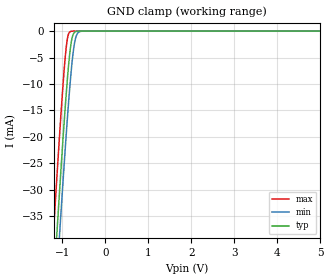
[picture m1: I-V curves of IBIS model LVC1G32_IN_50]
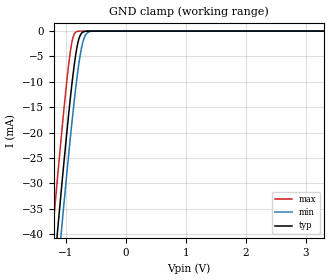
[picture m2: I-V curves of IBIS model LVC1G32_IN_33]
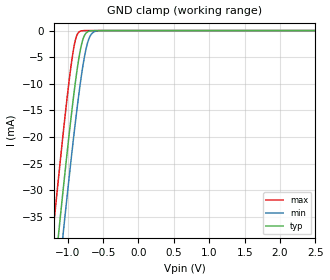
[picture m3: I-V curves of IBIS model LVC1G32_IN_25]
| TEXAS INSTRUMENTS INCORPORATED
| Standard Linear and Logic Group
| IBIS Model of SN74LVC1G32
| SINGLE 2-INPUT POSITIVE-OR GATE
| This file contains package information for the following:
|  SON 6-pin (DSF) package as [Component] LVC1G32_DSF
|  SOT 5-pin (DBV) package as [Component] LVC1G32_DBV
|  SOT 5-pin (DCK) package as [Component] LVC1G32_DCK
|  USON 6-pin (DRY) package as [Component] LVC1G32_DRY
|  NanoStar WCSP 5-pin (YEA) package as [Component] LVC1G32_YEA
|  NanoFree WCSP 5-pin (YZA) package as [Component] LVC1G32_YZA
|  NanoStar WCSP 5-pin (YEP) package as [Component] LVC1G32_YEP
|  NanoFree WCSP 5-pin (YZP) package as [Component] LVC1G32_YZP
| This device can be powered at the following Vccs:
|  5.0 volt Vcc
|  3.3 volt Vcc
|  2.5 volt Vcc
|  1.8 volt Vcc
| This file provides unique models under the [Model Selector] for each Vcc.
| For operation at a specific Vcc, select the appropriate model after each
| [Model Selector] keyword.
[IBIS Ver]   3.2
[Comment char]  |_char
[File Name]   sn74lvc1g32.ibs
[File Rev]   1.4 | d_die
[Date]   03/06/2014
[Source]
| Texas Instruments Incorporated.
| Analog-eLab Design Center, HPA
| 12500 TI Blvd
| Dallas, TX -75243
[Notes]   Revision History:
| The following is an IBIS list for the SN74LVC1G07.
| Please contact sllibis@ti.com with questions and
| comments concerning SLL IBIS models.
| - FILE REV HISTORY
| - 1.4 DSF package added 03/06/2014.
| - Rev 1.3. Added package component LVC1G32_DRY
| - 1.2 YEA, YEP, YZA, and YZP packages added on 05/18/04
| - As there is no power clamp diode in the Input Model,
|   we removed the Pwr Clamp table data from those Models.
| - Due to the fact that the Device is 5-V Input/Output
|   tolarent, the Model has some Non-Monotonic Warnings.
[Disclaimer]
| This model is designed as an aid for customers of Texas Instruments
| TI and its licensors and suppliers make no warranties, either expressed
| or implied, with respect to this  model, including the warranties of
| merchantability or fitness for a particular purpose.
| The model is provided solely on an "as is" basis. The entire risk as to
| its quality and performance is with the customer.
[Copyright]
(C) Copyright 2014 Texas Instruments Incorporated.All rights reserved.
| Component LVC1G32_DSF 6-pin SON
[Component]   LVC1G32_DSF
[Manufacturer]   Texas Instruments, Inc.
[Package]
|   typ   min   max
R_pkg   0.04185   0.03442   0.04904
L_pkg   0.42366nH   0.34696nH   0.51073nH
C_pkg   0.11042pF   0.10608pF   0.11529pF
[Pin]   signal_name   model_name   R_pin   L_pin   C_pin
1   A   LVC1G32_IN   0.04209   0.41329nH   0.10991pF
2   B   LVC1G32_IN   0.03442   0.34696nH   0.10608pF
3   GND   GND   0.04429   0.45885nH   0.11207pF
4   Y   LVC1G32_OUT   0.04904   0.51073nH   0.11529pF
5   nc   nc   0.00037   0.03788nH   0.07652pF
6   VCC   POWER   0.04377   0.44894nH   0.11182pF
| Component LVC1G32_DBV 5-pin SOT
[Component]   LVC1G32_DBV
[Manufacturer]   Texas Instruments, Inc.
[Package]
|   typ   min   max
R_pkg   2.500e-02   2.100e-02   2.900e-02
L_pkg   1.529e-09   1.312e-09   1.906e-09
C_pkg   1.560e-13   1.100e-13   2.400e-13
[Pin]   signal_name   model_name   R_pin   L_pin   C_pin
1   A   LVC1G32_IN   2.100e-02   1.511e-09   1.440e-13
2   B   LVC1G32_IN   2.300e-02   1.312e-09   1.380e-13
3   GND   GND   2.900e-02   1.906e-09   2.400e-13
4   Y   LVC1G32_OUT   2.600e-02   1.541e-09   1.500e-13
5   VCC   POWER   2.500e-02   1.374e-09   1.100e-13
| Component LVC1G32_DCK 5-pin SOT
[Component]   LVC1G32_DCK
[Manufacturer]   Texas Instruments, Inc.
[Package]
|   typ   min   max
R_pkg   2.000e-02   1.700e-02   2.500e-02
L_pkg   9.980e-10   8.810e-10   1.069e-09
C_pkg   1.460e-13   1.180e-13   2.050e-13
[Pin]   signal_name   model_name   R_pin   L_pin   C_pin
1   A   LVC1G32_IN   1.900e-02   1.069e-09   1.620e-13
2   B   LVC1G32_IN   1.800e-02   8.810e-10   1.210e-13
3   GND   GND   1.700e-02   1.031e-09   2.050e-13
4   Y   LVC1G32_OUT   2.000e-02   9.600e-10   1.240e-13
5   VCC   POWER   2.500e-02   1.049e-09   1.180e-13
| Component LVC1G32_YEA 5-pin NanoStar WCSP
[Component]   LVC1G32_YEA
[Manufacturer]   Texas Instruments, Inc.
[Package]
|   typ   min   max
R_pkg   0.001   0.001   0.001
L_pkg   0.021nH   0.021nH   0.021nH
C_pkg   0.046pF   0.045pF   0.047pF
[Pin]   signal_name   model_name   R_pin   L_pin   C_pin
1   A   LVC1G32_IN   0.001   0.021nH   0.046pF
2   B   LVC1G32_IN   0.001   0.021nH   0.047pF
3   GND   GND   0.001   0.021nH   0.046pF
4   Y   LVC1G32_OUT   0.001   0.021nH   0.045pF
5   VCC   POWER   0.001   0.021nH   0.045pF
| Component LVC1G32_YZA 5-pin NanoFree WCSP
[Component]   LVC1G32_YZA
[Manufacturer]   Texas Instruments, Inc.
[Package]
|   typ   min   max
R_pkg   0.001   0.001   0.001
L_pkg   0.021nH   0.021nH   0.021nH
C_pkg   0.046pF   0.045pF   0.047pF
[Pin]   signal_name   model_name   R_pin   L_pin   C_pin
1   A   LVC1G32_IN   0.001   0.021nH   0.046pF
2   B   LVC1G32_IN   0.001   0.021nH   0.047pF
3   GND   GND   0.001   0.021nH   0.046pF
4   Y   LVC1G32_OUT   0.001   0.021nH   0.045pF
5   VCC   POWER   0.001   0.021nH   0.045pF
| Component LVC1G32_YEP 5-pin NanoStar WCSP
[Component]   LVC1G32_YEP
[Manufacturer]   Texas Instruments, Inc.
[Package]
|   typ   min   max
R_pkg   0.001   0.001   0.001
L_pkg   0.021nH   0.021nH   0.021nH
C_pkg   0.046pF   0.045pF   0.047pF
[Pin]   signal_name   model_name   R_pin   L_pin   C_pin
1   A   LVC1G32_IN   0.001   0.021nH   0.046pF
2   B   LVC1G32_IN   0.001   0.021nH   0.047pF
3   GND   GND   0.001   0.021nH   0.046pF
4   Y   LVC1G32_OUT   0.001   0.021nH   0.045pF
5   VCC   POWER   0.001   0.021nH   0.045pF
| Component LVC1G32_YZP 5-pin NanoFree WCSP
[Component]   LVC1G32_YZP
[Manufacturer]   Texas Instruments, Inc.
[Package]
|   typ   min   max
R_pkg   0.001   0.001   0.001
L_pkg   0.021nH   0.021nH   0.021nH
C_pkg   0.046pF   0.045pF   0.047pF
[Pin]   signal_name   model_name   R_pin   L_pin   C_pin
1   A   LVC1G32_IN   0.001   0.021nH   0.046pF
2   B   LVC1G32_IN   0.001   0.021nH   0.047pF
3   GND   GND   0.001   0.021nH   0.046pF
4   Y   LVC1G32_OUT   0.001   0.021nH   0.045pF
5   VCC   POWER   0.001   0.021nH   0.045pF
| Component LVC1G32_DRY 6-pin USON
[Component]   LVC1G32_DRY
[Manufacturer]   Texas Instruments, Inc.
[Package]
|   typ   min   max
R_pkg   0.04988   0.00103   0.05683
L_pkg   0.40631n   0.01445n   0.47858n
C_pkg   0.10742p   0.07652p   0.11194p
[Pin]   signal_name   model_name   R_pin   L_pin   C_pin
1   A   LVC1G32_IN   0.05683   0.47858n   0.11194p
2   A   LVC1G32_IN   0.04686   0.38124n   0.10769p
3   GND   GND   0.05415   0.45213n   0.10986p
4   Y   LVC1G32_OUT   0.05132   0.42056n   0.10715p
5   NC   NC   0.00103   0.01445n   0.07652p
6   VCC   POWER   0.04843   0.39205n   0.10505p
| Model LVC1G32_IN
[Model Selector]   LVC1G32_IN
LVC1G32_IN_50   5.0 volt Vcc
LVC1G32_IN_33   3.3 volt Vcc
LVC1G32_IN_25   2.5 volt Vcc
LVC1G32_IN_18   1.8 volt Vcc
| Model LVC1G32_OUT
[Model Selector]   LVC1G32_OUT
LVC1G32_OUT_50   5.0 volt Vcc
LVC1G32_OUT_33   3.3 volt Vcc
LVC1G32_OUT_25   2.5 volt Vcc
LVC1G32_OUT_18   1.8 volt Vcc
| Models and submodels in the file (8): LVC1G32_IN_50 (Input), LVC1G32_IN_33 (Input), LVC1G32_IN_25 (Input), LVC1G32_IN_18 (Input), LVC1G32_OUT_50 (Output), LVC1G32_OUT_33 (Output), LVC1G32_OUT_25 (Output), LVC1G32_OUT_18 (Output)
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[Model]   LVC1G32_IN_50
Model_type  Input
Vinl =   1.35
Vinh =   3.85
| variable   typ   min   max
C_comp   3.21pF   2.52pF   4.35pF
[Temperature Range]   40   100   -40
| Ambient temperature   25   85   -40
[Voltage range]   5   4.5   5.5
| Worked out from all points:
|   GND clamp passes 1 mA (typ) near -0.77 V on its own axis
[GND Clamp]
| LVC1G32_IN_50
|   Voltage   I(typ)   I(min)   I(max)
-5V       -583.8mA   -590.8mA   -575.1mA
-1.21V    -48.93mA   -57.22mA   -38.3mA
-1.13V    -38.42mA   -46.71mA   -27.77mA
-1.07V    -30.71mA   -38.96mA   -20.13mA
-1.05V    -28.19mA   -36.42mA   -17.65mA
-915mV    -12.21mA   -19.95mA   -3.333mA
-870mV    -7.651mA   -14.9mA    -891.1uA
-815mV    -3.252mA   -9.299mA   -87.06uA
-770mV    -1.128mA   -5.445mA   -10.73uA
-705mV    -146.7uA   -1.723mA   -505nA
-575mV    -1.597uA   -52.97uA   -1.117nA
5V        9.69pA     12.83pA    9.218pA
[Model]   LVC1G32_IN_33
Model_type  Input
Vinl =   0.8
Vinh =   2.0
| variable   typ   min   max
C_comp   3.18pF   2.55pF   4.41pF
[Temperature Range]   40   100   -40
| Ambient temperature   25   85   -40
[Voltage range]   3.3   3   3.6
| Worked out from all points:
|   GND clamp passes 1 mA (typ) near -0.77 V on its own axis
[GND Clamp]
| LVC1G32_IN_33
|   Voltage   I(typ)   I(min)   I(max)
-5V       -583.8mA   -590.8mA   -575.1mA
-1.215V   -49.6mA    -57.88mA   -38.96mA
-1.14V    -39.72mA   -48.01mA   -29.07mA
-1.08V    -31.98mA   -40.25mA   -21.38mA
-1.06V    -29.44mA   -37.69mA   -18.89mA
-925mV    -13.29mA   -21.11mA   -4.122mA
-875mV    -8.124mA   -15.45mA   -1.065mA
-820mV    -3.579mA   -9.774mA   -109.4uA
-770mV    -1.128mA   -5.445mA   -10.73uA
-715mV    -205.4uA   -2.128mA   -808.5nA
-590mV    -2.7uA     -81.86uA   -2.255nA
3.3V      6.304pA    9.258pA    5.93pA
[Model]   LVC1G32_IN_25
Model_type  Input
Vinl =   0.7
Vinh =   1.7
| variable   typ   min   max
C_comp   3.17pF   2.55pF   4.29pF
[Temperature Range]   40   100   -40
| Ambient temperature   25   85   -40
[Voltage range]   2.5   2.3   2.7
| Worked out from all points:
|   GND clamp passes 1 mA (typ) near -0.77 V on its own axis
[GND Clamp]
| LVC1G32_IN_25
|   Voltage   I(typ)   I(min)   I(max)
-5V       -583.8mA   -590.8mA   -575.1mA
-1.205V   -48.27mA   -56.56mA   -37.63mA
-1.13V    -38.42mA   -46.71mA   -27.77mA
-1.07V    -30.71mA   -38.96mA   -20.13mA
-1.05V    -28.19mA   -36.42mA   -17.65mA
-955mV    -16.68mA   -24.66mA   -6.874mA
-885mV    -9.098mA   -16.55mA   -1.486mA
-830mV    -4.281mA   -10.75mA   -171.6uA
-780mV    -1.472mA   -6.227mA   -17.15uA
-710mV    -173.7uA   -1.918mA   -639nA
-645mV    -18.49uA   -387.7uA   -29.98nA
2.5V      4.713pA    7.577pA    4.389pA
